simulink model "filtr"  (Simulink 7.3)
settings: Solver=ode45  StartTime=0.0  StopTime=10.0  RelTol=1e-3
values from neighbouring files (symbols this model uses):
  Kp = om^2    (= 1)    [run.m]
  Kr = 2*zt*om    (= 0.28)    [run.m]

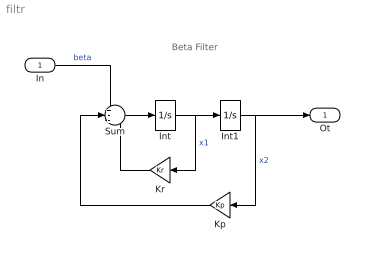
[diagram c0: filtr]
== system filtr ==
  note: Beta Filter
  In : Inport  OutDataType=fixdt(1, 16)  OutScaling=2^0
  Int : Integrator
  Int1 : Integrator
  Kp : Gain  Gain=Kp  ParameterDataType=sfix(16)  ParameterScaling=2^0  OutDataType=sfix(16)  OutScaling=2^0
  Kr : Gain  Gain=Kr  ParameterDataType=sfix(16)  ParameterScaling=2^0  OutDataType=sfix(16)  OutScaling=2^0
  Sum : Sum  Inputs=+--  OutDataType=sfix(16)  OutScaling=2^0
  Ot : Outport  OutDataType=fixdt(1, 16)  OutScaling=2^0
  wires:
  In/1 -> Sum/1  "beta"
  Int/1 -> Int1/1, Kr/1  "x1"
  Sum/1 -> Int/1
  Int1/1 -> Kp/1, Ot/1  "x2"
  Kr/1 -> Sum/3
  Kp/1 -> Sum/2
